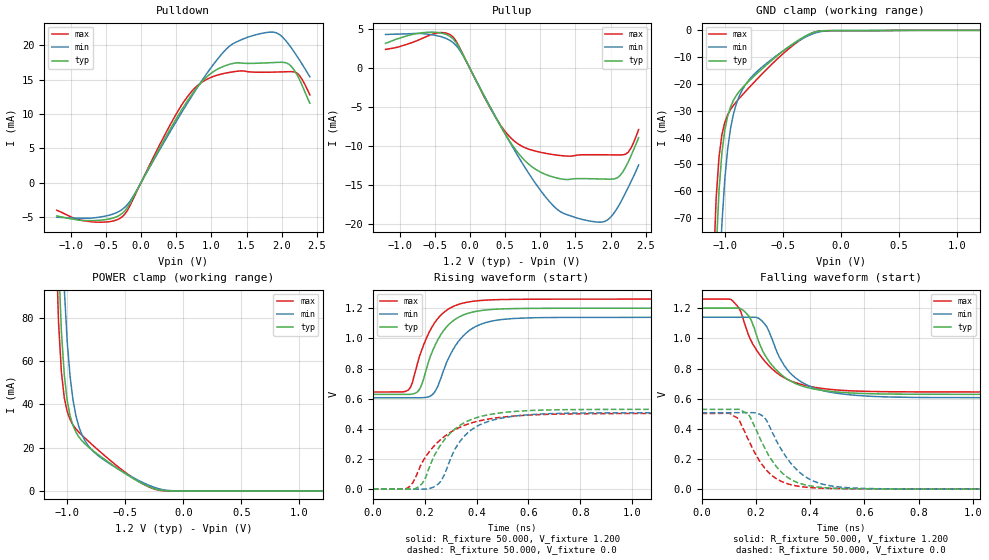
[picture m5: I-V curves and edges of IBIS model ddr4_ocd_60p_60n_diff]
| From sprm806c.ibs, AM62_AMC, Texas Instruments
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|   Model ddr4_ocd_60p_60n_diff
[Model] ddr4_ocd_60p_60n_diff
Model_type I/O
Polarity   Non-Inverting
Enable   Active-High
Vinl =  0.700V
Vinh =  0.900V
Vmeas =  0.600V
C_comp   2.366pF   2.354pF   2.430pF
[Model Spec]
Vinh   0.900V   0.820V   0.980V
Vinl   0.700V   0.620V   0.780V
Vmeas   0.600V   NA   NA
[Temperature Range]   25.000   0.125k   -40.000
[Voltage Range]   1.200V   1.140V   1.260V
[Pullup Reference]   1.200V   1.140V   1.260V
[Pulldown Reference]   0.0V   0.0V   0.0V
[C Comp Corner]
C_comp   2.354pF   2.366pF   2.430pF
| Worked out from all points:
|   slope of the pulldown table from 0 to 0.18 V, typ, clamps not added: 51.9 ohm
|   slope of the pullup table from 0 to 0.18 V, typ, clamps not added: 56.7 ohm
|   GND clamp passes 1 mA (typ) near -0.25 V on its own axis
|   POWER clamp passes 1 mA (typ) near -0.25 V on its own axis
|   rising waveform, R_fixture 50.000, V_fixture 1.200: 20-80 % time 91.9ps typ, 101ps min, 91.8ps max; typ from 0.629 V to 1.2 V
|   rising waveform, R_fixture 50.000, V_fixture 0.0: 20-80 % time 127ps typ, 113ps min, 155ps max; typ from 0.002 V to 0.53 V
|   falling waveform, R_fixture 50.000, V_fixture 1.200: 20-80 % time 116ps typ, 115ps min, 129ps max; typ from 1.2 V to 0.629 V
|   falling waveform, R_fixture 50.000, V_fixture 0.0: 20-80 % time 105ps typ, 115ps min, 98.9ps max; typ from 0.53 V to 0.002 V
[Pulldown]
|Voltage   I(typ)   I(min)   I(max)
-1.2V     -4.862mA   -5.049mA   -4.03mA
-718mV    -5.546mA   -5.182mA   -5.698mA
-272mV    -4.526mA   -3.943mA   -5.015mA
-124mV    -2.402mA   -2.19mA    -2.644mA
396mV     7.455mA    7.097mA    8.073mA
693mV     12.41mA    12.13mA    12.96mA
990mV     15.88mA    16.67mA    15.3mA
1.324V    17.39mA    20.32mA    16.16mA
1.918V    17.5mA     21.83mA    16.1mA
2.14V     16.88mA    19.56mA    16.15mA
2.252V    15.04mA    17.86mA    15.6mA
2.4V      11.56mA    15.4mA     12.77mA
[Pullup]
|Voltage   I(typ)   I(min)   I(max)
-1.2V     3.216mA    4.353mA    2.435mA
-532mV    4.66mA     4.317mA    4.393mA
-346mV    4.399mA    3.876mA    4.56mA
-198mV    3.349mA    2.954mA    3.533mA
247mV     -4.328mA   -4.234mA   -4.391mA
544mV     -9.04mA    -9.105mA   -8.565mA
878mV     -12.6mA    -14.04mA   -10.49mA
1.324V    -14.24mA   -18.59mA   -11.23mA
1.955V    -14.23mA   -19.49mA   -11.1mA
2.103V    -14.02mA   -17.85mA   -11.12mA
2.252V    -12.02mA   -15.29mA   -10.76mA
2.4V      -8.904mA   -12.4mA    -7.854mA
[GND_clamp]
|Voltage   I(typ)   I(min)   I(max)
-1.2V     -396.3mA   -450.8mA   -370.5mA
-1.1V     -118.3mA   -172.8mA   -91.44mA
-1.075V   -83.02mA   -129.3mA   -63.08mA
-1.05V    -59.94mA   -96.19mA   -47.32mA
-1.025V   -45.76mA   -72.24mA   -38.96mA
-1V       -37.22mA   -55.56mA   -34.32mA
-975mV    -31.95mA   -44.18mA   -31.47mA
-925mV    -26.07mA   -31.12mA   -27.96mA
-775mV    -18.22mA   -17.64mA   -20.64mA
-425mV    -5.392mA   -5.54mA    -6.048mA
-175mV    -232.3uA   -493.9uA   -237.3uA
1.2V      0A         0A         0A
[POWER_clamp]
|Voltage   I(typ)   I(min)   I(max)
-1.2V     594.8mA    732.7mA    623.3mA
-1.1V     157.8mA    248.4mA    121.5mA
-1.075V   106.2mA    179.2mA    77.8mA
-1.05V    73.23mA    128.5mA    54.67mA
-1.025V   53.34mA    92.89mA    42.85mA
-1V       41.61mA    68.72mA    36.57mA
-975mV    34.56mA    52.6mA     32.87mA
-925mV    27.12mA    34.66mA    28.61mA
-825mV    20.64mA    21.33mA    23.28mA
-675mV    14.44mA    14mA       16.15mA
-200mV    388.1uA    876.1uA    237.2uA
1.2V      0A         0A         0A
[Ramp]
| variable   typ   min   max
dV/dt_r   0.317/0.126n   0.335/0.124n   0.300/0.156n
dV/dt_f   0.342/0.115n   0.351/0.123n   0.369/0.128n
R_load = 60.000
[Rising Waveform]
R_fixture= 50.000
V_fixture= 1.200
V_fixture_min= 1.140
V_fixture_max= 1.260
|time   V(typ)   V(min)   V(max)
0s        629.2mV    606.9mV    645mV
140ps     629mV      607mV      663.4mV
182ps     667.6mV    606.7mV    889.9mV
225ps     893.6mV    620.3mV    1.064V
249ps     983.8mV    675.9mV    1.128V
291ps     1.088V     864mV      1.193V
337ps     1.145V     994.9mV    1.228V
397ps     1.178V     1.078V     1.247V
617ps     1.198V     1.136V     1.259V
3ns       1.2V       1.14V      1.26V
[Rising Waveform]
R_fixture= 50.000
V_fixture= 0.0
V_fixture_min= 0.0
V_fixture_max= 0.0
|time   V(typ)   V(min)   V(max)
0s        1.981mV    2.204mV    3.443mV
142ps     1.955mV    2.193mV    19.63mV
190ps     38.41mV    2.189mV    177.8mV
236ps     216.8mV    17.39mV    286.4mV
261ps     292.9mV    52.67mV    329mV
287ps     351.3mV    144mV      364.4mV
316ps     398.5mV    264.5mV    394.5mV
356ps     444mV      358.9mV    425.8mV
507ps     510mV      475.3mV    480mV
3ns       530.1mV    508mV      503.2mV
[Falling Waveform]
R_fixture= 50.000
V_fixture= 1.200
V_fixture_min= 1.140
V_fixture_max= 1.260
|time   V(typ)   V(min)   V(max)
0s        1.2V       1.14V      1.26V
114ps     1.2V       1.14V      1.25V
144ps     1.197V     1.14V      1.18V
174ps     1.148V     1.14V      1.018V
212ps     971.6mV    1.131V     896.7mV
249ps     845.4mV    1.042V     817.3mV
323ps     722.4mV    775.8mV    722.7mV
463ps     651.5mV    647.3mV    664.2mV
813ps     629.8mV    608.4mV    645.4mV
3ns       629.2mV    606.9mV    645mV
[Falling Waveform]
R_fixture= 50.000
V_fixture= 0.0
V_fixture_min= 0.0
V_fixture_max= 0.0
|time   V(typ)   V(min)   V(max)
0s        530mV      508mV      503.2mV
102ps     530mV      508mV      503.5mV
133ps     530.4mV    508mV      471.4mV
175ps     490.4mV    508mV      320mV
223ps     309.8mV    488.9mV    163.5mV
305ps     95.86mV    232.8mV    44.99mV
359ps     42.3mV     116.3mV    20.79mV
429ps     15.88mV    43.9mV     9.528mV
639ps     3.32mV     5.177mV    4.2mV
3ns       1.98mV     2.197mV    3.443mV
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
